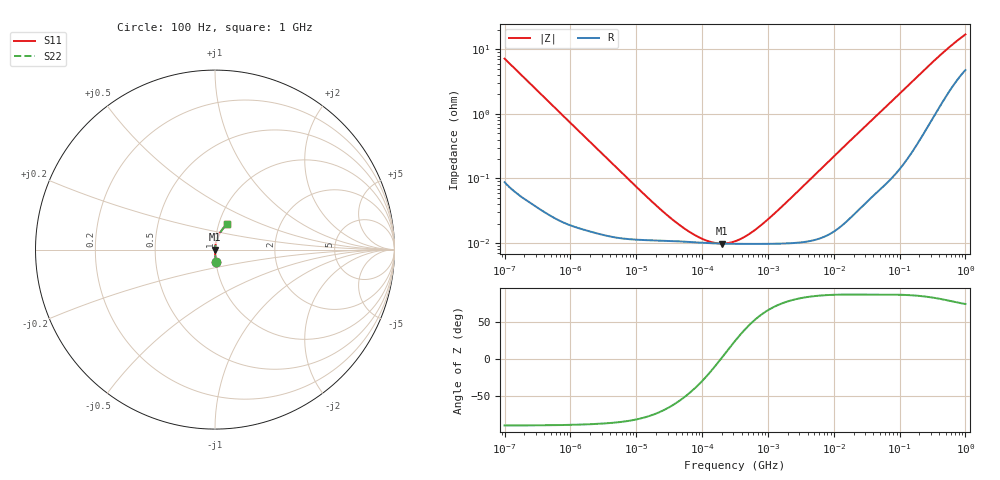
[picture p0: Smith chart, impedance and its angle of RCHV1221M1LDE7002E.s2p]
! RCHV1221M1LDE7002E  S-PARAMETER MODEL  (AEC-Q200 qualified)
! Model Generated by ELNA Corporation (http://www.ty-top.com)
! Version 1.0
! ELNA Control No.240229
! Copyright (c) 2024 ELNA CO.,LTD. All Rights Reserved.
! Products Name : CONDUCTIVE POLYMER HYBRID ALUMINUM ELECTROLYTIC CAPACITORS
! Characteristics :
!  Capacitance  :  220uF  ,  Rated voltage  :  10V
!  Operating Temp. Range  :  -55 to +105 degC  ,  Endurance  :  10000hr at 105 degC
!  Dimension D  :  6.3mm  ,  Dimension L  :  7.7mm
! Frequency Range : 100Hz - 1GHz
! External Node Assignments :
!  1  o---| |---o  2
# MHz S RI R 50
!Freq[MHz].  S11 Real  S11 Imag  S21 Real  S21 Imag  S12 Real  S12 Imag  S22 Real  S22 Imag
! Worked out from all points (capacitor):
!   401 points, 100 Hz to 1 GHz, reference 50 ohm
!   read as one part in series: C = 222 uF near 108 Hz
!   lowest |Z| = 9.83 mohm at 203 kHz (marker M1)
!   series resonance near 193.1 kHz, so ESL is about 3.1 nH
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0.0001  0.00596 -0.0711  0.994 0.0711  0.994 0.0711  0.00596 -0.0711
0.000113  0.00477 -0.0631  0.9952 0.0631  0.9952 0.0631  0.00477 -0.0631
0.000309  0.000899 -0.0232  0.9991 0.0232  0.9991 0.0232  0.000899 -0.0232
0.001488  0.000188 -0.00489  0.9998 0.00489  0.9998 0.00489  0.000188 -0.00489
0.010292  0.000113 -0.000715  0.9999 0.000715  0.9999 0.000715  0.000113 -0.000715
0.022131  0.00011 -0.000332  0.9999 0.000332  0.9999 0.000332  0.00011 -0.000332
0.043904  0.000107 -0.000164  0.9999 0.000164  0.9999 0.000164  0.000107 -0.000164
0.080353  0.000103 -8.06e-05  0.9999 8.06e-05  0.9999 8.06e-05  0.000103 -8.06e-05
0.106537  0.000101 -5.18e-05  0.9999 5.18e-05  0.9999 5.18e-05  0.000101 -5.18e-05
0.135675  9.97e-05 -2.99e-05  0.9999 2.99e-05  0.9999 2.99e-05  9.97e-05 -2.99e-05
0.203002  9.82e-05 4.21e-06  0.9999 -4.21e-06  0.9999 -4.21e-06  9.82e-05 4.21e-06
0.258523  9.77e-05 2.5e-05  0.9999 -2.5e-05  0.9999 -2.5e-05  9.77e-05 2.5e-05
0.316228  9.74e-05 4.34e-05  0.9999 -4.34e-05  0.9999 -4.34e-05  9.74e-05 4.34e-05
0.492606  9.72e-05 9.15e-05  0.9999 -9.15e-05  0.9999 -9.15e-05  9.72e-05 9.15e-05
0.798914  9.72e-05 0.000165  0.9999 -0.000165  0.9999 -0.000165  9.72e-05 0.000165
1.522299  9.82e-05 0.000329  0.9999 -0.000329  0.9999 -0.000329  9.82e-05 0.000329
4.704354  0.00011 0.00103  0.9999 -0.00103  0.9999 -0.00103  0.00011 0.00103
69.9842  0.00113 0.0144  0.9989 -0.0144  0.9989 -0.0144  0.00113 0.0144
176.8072  0.00441 0.0355  0.9956 -0.0355  0.9956 -0.0355  0.00441 0.0355
395.8221  0.0178 0.0745  0.9822 -0.0745  0.9822 -0.0745  0.0178 0.0745
668.3439  0.0407 0.112  0.9593 -0.112  0.9593 -0.112  0.0407 0.112
1000  0.0679 0.1446  0.9321 -0.1446  0.9321 -0.1446  0.0679 0.1446
